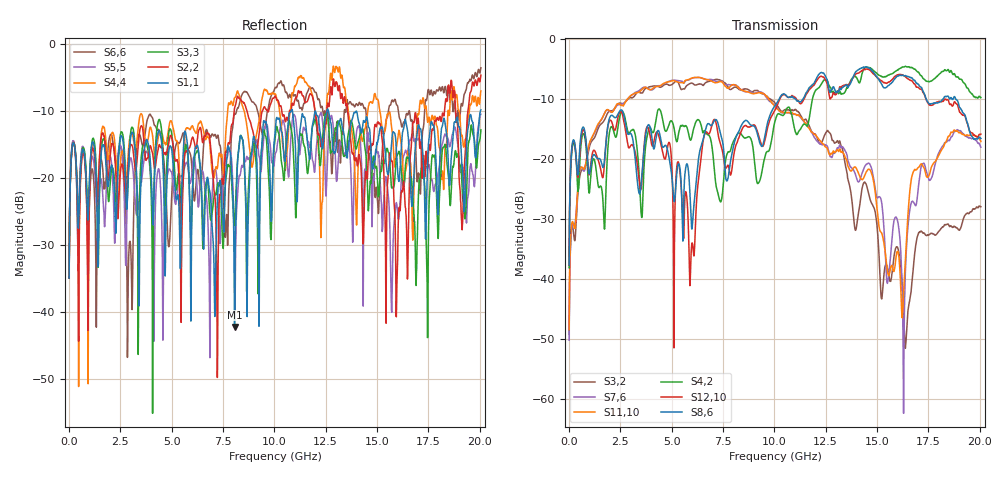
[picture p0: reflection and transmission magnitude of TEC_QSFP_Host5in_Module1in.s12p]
!!  This file represents Tyco Electronics parts only.  Due to internal design and materials, it should not  !!
!!  be used for products manufactured by companies other than Tyco Electronics.  !!
!! FILE NAME: TEC_QSFP_Host5in_Module1in.s12p
!! PART DESCRIPTION: Tyco Electronics QSFP P/N 1761987-9
!! PCB DESCRIPTION: Host Board FR4 with 5 inch microstrip, Module Board FR4 with 1.5 inch microstrip
!! FILE DESCRIPTION: 12 Port, S-Parameter, Measured Channel
!! FILE REVISION: Revision 2, 3/11/2008
!! FILE FREQUENCY RANGE: DC to 20.05 GHz in 12.50 MHz frequency steps
!! PORT DEFINITIONS:
!! Port  1  ----->  Host	Pin 14, RX3+	Module  <-----  Port  2
!! Port  3  ----->  Host	Pin 15, RX3-	Module  <-----  Port  4
!! Port  5  ----->  Host	Pin 21, RX2-	Module  <-----  Port  6
!! Port  7  ----->  Host	Pin 22, RX2+	Module  <-----  Port  8
!! Port  9  ----->  Host	Pin 24, RX4-	Module  <-----  Port  10
!! Port  11  ----->  Host	Pin 25, RX4+	Module  <-----  Port  12
# HZ S MA R 50.00
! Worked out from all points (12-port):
!   1604 points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, 12.5 MHz to 20.05 GHz, reference 50 ohm
!   strongest paths, dB at 12.5 MHz, 5.025 GHz, 10.04 GHz, 15.05 GHz, 20.05 GHz:
!     S8,6: -37.6, -23.4, -11.1, -6.6, -16.6
!     S12,10: -37.6, -22.4, -11.8, -6.5, -15.8
!     S4,2: -38.1, -13.8, -13.6, -5.9, -9.7
!     S11,10: -48.4, -7.0, -11.3, -30.0, -17.1
!     S7,6: -50.1, -6.9, -11.1, -26.3, -18.0
!     S3,2: -49.1, -7.6, -10.7, -33.4, -27.9
!   lowest |S11| = -42.3 dB at 8.062 GHz (marker M1), VSWR 1.02, Z = 49.6 - j0.657 ohm
!   |S11| at or under -10 dB: start of sweep to 10.82 GHz; 10.88 GHz to 12.56 GHz (1.681 GHz wide, 14.3 % of centre); 12.63 GHz to 20.03 GHz (7.406 GHz wide, 45.3 % of centre)
